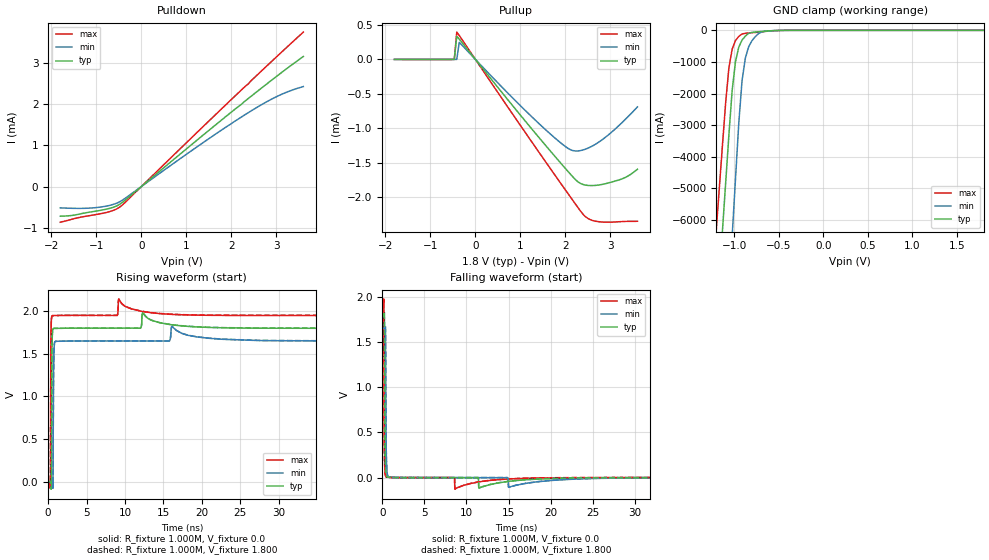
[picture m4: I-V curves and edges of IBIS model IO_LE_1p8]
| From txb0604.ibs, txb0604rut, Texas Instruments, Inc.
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[Model] IO_LE_1p8
Model_type 3-state
Polarity   Non-Inverting
Enable   Active-High
Vmeas =  0.900V
Cref =  15.000pF
Rref =  1.000M
Vref =  0.0V
C_comp   3.790pF   3.490pF   3.980pF
[Temperature Range]   27.000   0.125k   -40.000
[Voltage Range]   1.800V   1.650V   1.950V
[Pullup Reference]   1.800V   1.650V   1.950V
[Pulldown Reference]   0.0V   0.0V   0.0V
[POWER Clamp Reference]   1.800V   1.650V   1.950V
[GND Clamp Reference]   0.0V   0.0V   0.0V
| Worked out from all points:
|   slope of the pulldown table from 0 to 0.27 V, typ, clamps not added: 1.09 kohm
|   slope of the pullup table from 0 to 0.27 V, typ, clamps not added: 1.22 kohm
|   GND clamp passes 1 mA (typ) near -0.43 V on its own axis
|   rising waveform, R_fixture 1.000M, V_fixture 0.0: 20-80 % time 52.3ps typ, 64.8ps min, 47.6ps max; typ from 0 V to 1.8 V
|   rising waveform, R_fixture 1.000M, V_fixture 1.800: 20-80 % time 52.4ps typ, 65ps min, 47.6ps max; typ from 0.002 V to 1.8 V
|   falling waveform, R_fixture 1.000M, V_fixture 0.0: 20-80 % time 61.2ps typ, 63.5ps min, 48.7ps max; typ from 1.8 V to 0 V
|   falling waveform, R_fixture 1.000M, V_fixture 1.800: 20-80 % time 61.1ps typ, 63.2ps min, 48.6ps max; typ from 1.8 V to 0.002 V
[Pulldown]
|Voltage   I(typ)   I(min)   I(max)
-1.8V     -716uA     -514.4uA   -861.2uA
-1.525V   -695.5uA   -525.3uA   -785.1uA
-1.03V    -597.1uA   -510.5uA   -680.3uA
-700mV    -525.6uA   -453.9uA   -603.9uA
-480mV    -428.1uA   -366.9uA   -496.2uA
1.335V    1.212mA    1.036mA    1.412mA
2.325V    2.087mA    1.754mA    2.441mA
2.71V     2.418mA    2.006mA    2.84mA
3.04V     2.696mA    2.195mA    3.176mA
3.315V    2.922mA    2.321mA    3.454mA
3.6V      3.148mA    2.42mA     3.739mA
[Pullup]
|Voltage   I(typ)   I(min)   I(max)
-1.8V     20.9nA     9.445nA    96.61nA
-470mV    220.1nA    14.93nA    1.26uA
-415mV    335.7uA    239.8nA    396.7uA
-360mV    294.6uA    247.4uA    347.4uA
1.345V    -1.081mA   -889.6uA   -1.284mA
1.895V    -1.504mA   -1.21mA    -1.797mA
2.17V     -1.708mA   -1.323mA   -2.05mA
2.28V     -1.776mA   -1.327mA   -2.151mA
2.445V    -1.823mA   -1.301mA   -2.281mA
2.61V     -1.829mA   -1.251mA   -2.337mA
3.27V     -1.729mA   -907.6uA   -2.351mA
3.6V      -1.593mA   -688.5uA   -2.347mA
[GND_clamp]
|Voltage   I(typ)   I(min)   I(max)
-1.8V     -34.36A    -44.21A    -29.4A
-1.208V   -9.521A    -15.48A    -6.558A
-1.171V   -7.969A    -13.69A    -5.131A
-1.134V   -6.417A    -11.89A    -3.704A
-1.06V    -3.312A    -8.299A    -1.19A
-1.023V   -1.893A    -6.504A    -593mA
-986mV    -994.4mA   -4.708A    -323.1mA
-949mV    -530.7mA   -2.941A    -190.7mA
-912mV    -308.1mA   -1.586A    -114.8mA
-838mV    -95.13mA   -519.5mA   -83.45mA
-653mV    -26.56mA   -29.86mA   -34.54mA
1.8V      0A         0A         0A
[Ramp]
| variable   typ   min   max
dV/dt_r   1.079/55.634p   0.988/67.062p   1.169/45.757p
dV/dt_f   1.079/55.902p   0.989/66.434p   1.169/46.608p
R_load = 1.000M
[Rising Waveform]
R_fixture= 1.000M
V_fixture= 0.0
V_fixture_min= 0.0
V_fixture_max= 0.0
|time   V(typ)   V(min)   V(max)
0s        337.1nV    150.9uV    176.4nV
290ps     -105.5uV   84.34uV    -76.98mV
340ps     3.692mV    -29.18uV   1.274V
400ps     -85.58mV   -198.9uV   1.851V
490ps     1.49V      1.56mV     1.941V
610ps     1.783V     -74.99mV   1.947V
710ps     1.796V     1.309V     1.948V
870ps     1.798V     1.64V      1.948V
9.19ns    1.8V       1.65V      2.141V
120ns     1.798V     1.648V     1.948V
[Rising Waveform]
R_fixture= 1.000M
V_fixture= 1.800
V_fixture_min= 1.650
V_fixture_max= 1.950
|time   V(typ)   V(min)   V(max)
0s        1.961mV    2.23mV     1.829mV
290ps     1.857mV    2.163mV    -75.1mV
340ps     5.672mV    2.05mV     1.276V
400ps     -83.61mV   1.882mV    1.852V
490ps     1.491V     3.661mV    1.941V
610ps     1.784V     -72.86mV   1.947V
710ps     1.796V     1.31V      1.948V
870ps     1.798V     1.64V      1.948V
9.19ns    1.8V       1.65V      2.141V
120ns     1.8V       1.65V      1.95V
[Falling Waveform]
R_fixture= 1.000M
V_fixture= 0.0
V_fixture_min= 0.0
V_fixture_max= 0.0
|time   V(typ)   V(min)   V(max)
0s        1.798V     1.648V     1.948V
180ps     1.792V     1.648V     1.956V
250ps     1.814V     1.644V     318mV
300ps     626.9mV    1.633V     103.6mV
380ps     113.5mV    1.631V     23.51mV
410ps     62.42mV    1.088V     14.06mV
490ps     20.24mV    202.9mV    7.07mV
670ps     5.306mV    14.99mV    3.791mV
8.64ns    10.56uV    24.17uV    -127.3mV
120ns     26.79uV    194.1uV    15.29uV
[Falling Waveform]
R_fixture= 1.000M
V_fixture= 1.800
V_fixture_min= 1.650
V_fixture_max= 1.950
|time   V(typ)   V(min)   V(max)
0s        1.8V       1.65V      1.95V
180ps     1.794V     1.651V     1.958V
250ps     1.816V     1.646V     318.6mV
300ps     628.6mV    1.635V     96.6mV
380ps     113.6mV    1.634V     23.62mV
410ps     62.52mV    1.089V     14.12mV
490ps     20.3mV     203.4mV    7.162mV
670ps     5.342mV    15.05mV    3.829mV
8.64ns    40.53uV    55.24uV    -127.2mV
120ns     1.987mV    2.273mV    1.844mV
